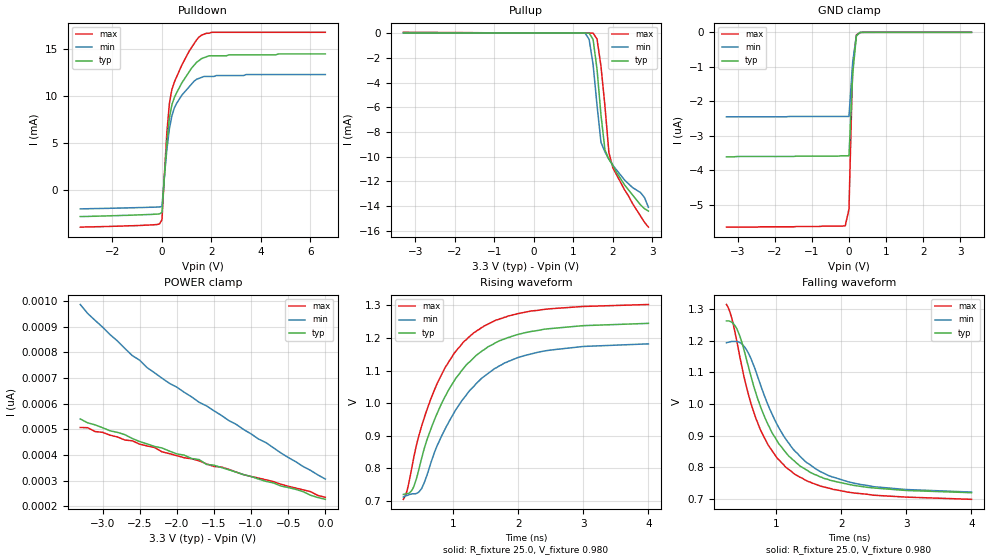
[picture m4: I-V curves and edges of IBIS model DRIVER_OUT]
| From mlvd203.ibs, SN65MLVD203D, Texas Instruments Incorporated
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|   Driver Output Model
[Model]   DRIVER_OUT
Model_type   3-state
| Signals   Y,Z
Vmeas = 1.0V   |Reference voltage for timing measurements
Cref = 3pF   |Timing specification test load capacitance value
Rref = 25   |Note: 50 Ohm load; single ended configuration
| variable   typ   min   max
C_comp   1.0pF   NA   NA
|   typ   min   max
[Temperature Range]   25.0   85   -40
[Voltage range]   3.3V   3.0V   3.6V
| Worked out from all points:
|   slope of the pulldown table from 0 to 0.495 V, typ, clamps not added: 40.6 ohm
|   rising waveform, R_fixture 25.0, V_fixture 0.980: 20-80 % time 811ps typ, 874ps min, 754ps max; typ from 0.719 V to 1.25 V
|   falling waveform, R_fixture 25.0, V_fixture 0.980: 20-80 % time 705ps typ, 765ps min, 647ps max; typ from 1.26 V to 0.719 V
[Pulldown]
|   Voltage   I(typ)   I(min)   I(max)
-3.3V     -2.82mA    -2mA       -3.95mA
-100mV    -2.54mA    -1.8mA     -3.61mA
0V        -2.38mA    -1.74mA    -3.16mA
100mV     1.47mA     1.47mA     1.74mA
200mV     5.06mA     4.38mA     6.17mA
300mV     7.65mA     6.52mA     9.22mA
400mV     9.08mA     7.9mA      10.7mA
500mV     9.85mA     8.75mA     11.5mA
800mV     11.4mA     10.1mA     13.3mA
1.5V      13.8mA     11.9mA     16.3mA
2V        14.3mA     12.1mA     16.8mA
6.6V      14.5mA     12.3mA     16.8mA
[Pullup]
|   Voltage   I(typ)   I(min)   I(max)
| Note that the[Pullup]voltage table is referenced to Vcc
| and is calculated using Vtable=Vcc - Vmeasured.
-3.3V     14.9uA     12.2uA     60uA
1.3V      -626nA     -14.9uA    -338nA
1.4V      -5.4uA     -510uA     -704nA
1.5V      -514uA     -2.53mA    -1.95uA
1.6V      -2.93mA    -5.84mA    -486uA
1.7V      -6.63mA    -8.84mA    -2.69mA
1.8V      -9.45mA    -9.61mA    -5.9mA
1.9V      -10.2mA    -10.2mA    -9.66mA
2V        -10.7mA    -10.7mA    -10.9mA
2.3V      -12.3mA    -11.9mA    -12.7mA
2.7V      -13.9mA    -12.9mA    -14.8mA
2.9V      -14.4mA    -14.1mA    -15.7mA
[GND_clamp]
|   Voltage   I(typ)   I(min)   I(max)
-3.3V     -3.61uA    -2.45uA    -5.65uA
-100mV    -3.58uA    -2.44uA    -5.61uA
0V        -3.58uA    -2.44uA    -5.13uA
100mV     -1.22uA    -868nA     -968nA
200mV     -103nA     -88.8nA    -75.4nA
300mV     -3.43nA    -5.37nA    -2.64nA
400mV     -48.6pA    -393pA     -16.8pA
3.3V      227pA      355pA      213pA
[Power_clamp]
| Note that the[POWER_clamp]voltage table is referenced to Vcc
| and is calculated using Vtable=Vcc - Vmeasured.
|   Voltage   I(typ)   I(min)   I(max)
-3.3V     540pA      986pA      507pA
-3.2V     525pA      951pA      506pA
-3.1V     517pA      924pA      491pA
-2.6V     464pA      787pA      455pA
-2.5V     452pA      769pA      442pA
-2.4V     443pA      740pA      435pA
-2.2V     427pA      699pA      412pA
-1.7V     382pA      605pA      377pA
-1.6V     363pA      591pA      365pA
-400mV    266pA      374pA      271pA
-200mV    243pA      340pA      257pA
0V        227pA      306pA      235pA
[Ramp]
|   typ   min   max
dV/dt_r   0.324/818ps   0.290/885ps   0.373/760ps
dV/dt_f   0.324/718ps   0.290/789ps   0.372/659ps
R_load = 25ohm  | Note: The measurement is single-ended with 25ohm
|   to ground.
[Rising Waveform]
R_fixture = 25.0
V_fixture = 0.980
V_fixture_min = 0.950
V_fixture_max = 1.000
C_fixture = 0p
L_fixture = 0n
|   V(typ)   V(min)   V(max)
240ps     719mV      711mV      704mV
300ps     722mV      716mV      733mV
380ps     735mV      721mV      812mV
520ps     830mV      737mV      929mV
760ps     969mV      870mV      1.061V
1.04ns    1.075V     978mV      1.158V
1.32ns    1.139V     1.051V     1.216V
1.78ns    1.196V     1.122V     1.263V
2.3ns     1.223V     1.156V     1.285V
4ns       1.245V     1.182V     1.303V
[Falling Waveform]
R_fixture = 25.0
V_fixture = 0.980
V_fixture_min = 0.950
V_fixture_max = 1.000
C_fixture = 0p
L_fixture = 0n
|   V(typ)   V(min)   V(max)
240ps     1.263V     1.194V     1.315V
320ps     1.259V     1.198V     1.273V
440ps     1.218V     1.195V     1.155V
580ps     1.116V     1.16V      1.028V
680ps     1.042V     1.11V      961mV
920ps     917mV      977mV      858mV
1.16ns    844mV      886mV      798mV
1.62ns    775mV      793mV      745mV
2.1ns     746mV      754mV      721mV
4ns       719mV      721mV      698mV
